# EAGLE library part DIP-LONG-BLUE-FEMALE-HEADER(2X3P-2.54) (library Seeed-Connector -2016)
320030066
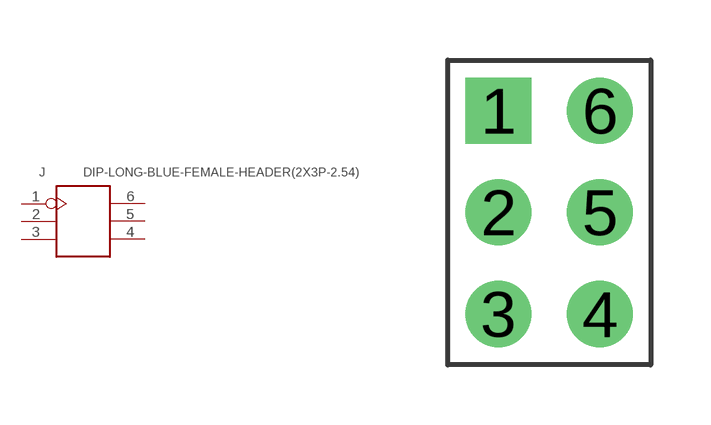
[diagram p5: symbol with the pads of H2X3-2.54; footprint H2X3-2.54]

Designator prefix J

## DIP-LONG-BLUE-FEMALE-HEADER(2X3P-2.54) (VALUE: 2x3p-2.54)  [H2X3-2.54]
1  1
2  2
3  3
4  4
5  5
6  6

## Footprint H2X3-2.54 (pad centres in mm)
drill 0.889 pad 1.651 square: 1 -1.27,2.54
drill 0.889 pad 1.651: 2 -1.27,0; 3 -1.27,-2.54; 4 1.27,-2.54; 5 1.27,0; 6 1.27,2.54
